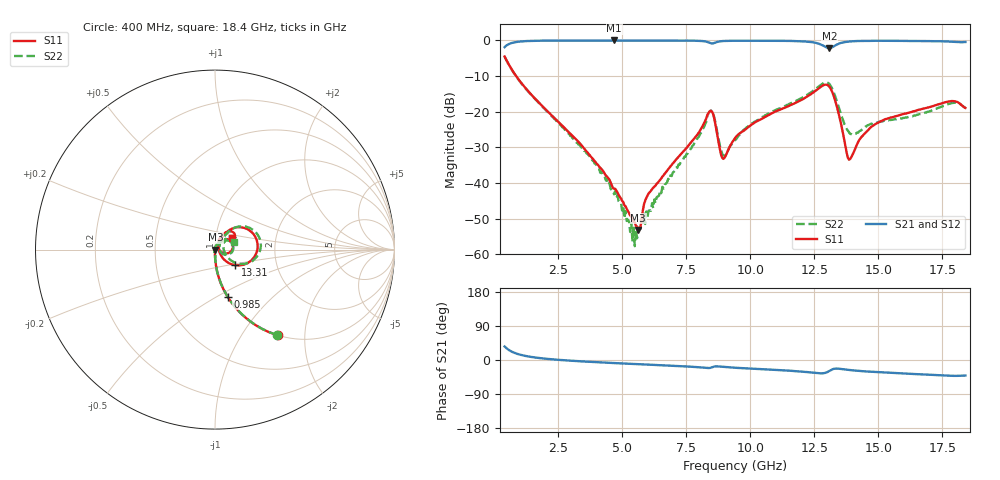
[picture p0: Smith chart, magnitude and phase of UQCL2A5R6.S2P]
! AVX Corporation
! Date:  10/27/06
! Part No:  UQCL2A5R6
! Description:  Ultra Low ESR Microwave capacitors
! Mounting Orientation:  Horizontal
# GHZ S DB R 50
! Freq  |S11|  S11 Ph  |S21|  S21 Ph  |S12|  S12 Ph  |S22|  S22 Ph
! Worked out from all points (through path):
!   401 points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, 400 MHz to 18.4 GHz, reference 50 ohm
!   highest |S21| = -0.03 dB at 4.675 GHz (marker M1); lowest = -2.2 dB at 13.09 GHz (marker M2)
!   group delay of S21, straight-line fit = 7.99 ps
!   lowest |S11| = -53.2 dB at 5.62 GHz (marker M3), VSWR 1.00, Z = 50.2 + j0.0239 ohm
!   |S11| at or under -10 dB: 849 MHz to end of sweep
!   |S22| runs from -57.7 to -4.6 dB; largest |S21 - S12| = 0.0022
!   S11 on the Smith chart (normalised r, x): 400 MHz: 1.00, -1.47; 985 MHz: 0.99, -0.56; 13.31 GHz: 1.23, -0.22; 18.4 GHz: 1.19, +0.15
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0.4  -4.54 -53.7  -1.91 35.7  -1.91 35.7  -4.61 -54.0
0.985  -11.34 -75.1  -0.35 14.4  -0.34 14.4  -11.42 -75.2
3.415  -29.49 -90.8  -0.04 -3.6  -0.03 -3.6  -30.14 -89.6
4.675  -41.58 -78.5  -0.03 -8.0  -0.03 -8.1  -43.16 -95.3
5.395  -50.27 -37.6  -0.04 -10.4  -0.04 -10.4  -56.44 -142.4
5.62  -53.17 6.2  -0.05 -11.1  -0.04 -11.1  -53.09 163.1
5.935  -44.19 46.9  -0.05 -11.9  -0.04 -12.0  -47.99 113.0
6.43  -39.50 51.4  -0.04 -13.5  -0.04 -13.5  -43.55 89.5
8.005  -25.65 53.6  -0.14 -19.2  -0.13 -19.2  -26.79 58.1
8.41  -19.91 26.8  -0.67 -21.0  -0.67 -21.0  -20.00 21.9
8.545  -20.68 -4.2  -0.85 -18.2  -0.85 -18.2  -20.38 -9.2
8.905  -33.01 6.9  -0.21 -18.1  -0.21 -18.1  -31.95 -5.9
9.4  -27.43 57.6  -0.11 -20.5  -0.11 -20.5  -27.96 46.6
10.075  -23.50 60.5  -0.09 -23.0  -0.09 -23.0  -23.22 54.2
12.415  -14.84 43.6  -0.52 -33.2  -0.52 -33.2  -14.37 42.6
13.09  -13.03 -10.6  -2.18 -28.6  -2.18 -28.6  -12.26 -6.4
13.315  -16.95 -37.8  -1.43 -22.9  -1.43 -22.9  -15.69 -29.1
13.855  -33.47 2.9  -0.33 -26.2  -0.33 -26.3  -25.81 -7.0
14.665  -24.64 67.6  -0.15 -30.7  -0.15 -30.8  -23.55 38.9
15.43  -21.75 65.0  -0.13 -33.8  -0.12 -33.8  -22.27 42.7
17.77  -17.12 45.0  -0.34 -41.4  -0.34 -41.5  -17.77 33.9
18.4  -18.96 34.5  -0.46 -41.1  -0.45 -41.1  -18.88 20.8
